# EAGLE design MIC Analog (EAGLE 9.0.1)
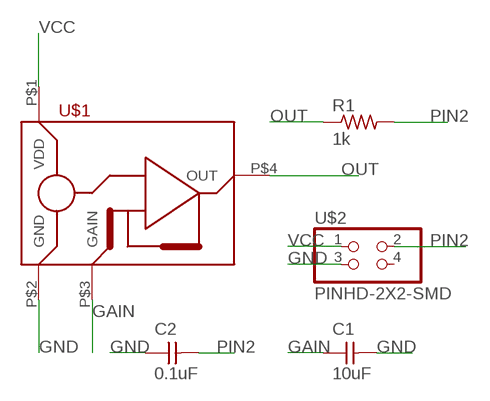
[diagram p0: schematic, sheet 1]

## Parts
C1  10uF  CAP-UNPOLARIZEDFAB  [C1206FAB]
C2  0.1uF  CAP-UNPOLARIZEDFAB  [C1206FAB]
R1  1k  RES-US1206FAB  [R1206FAB]
U$1  MEMS_MIC_SPU0414HR5H-SB  [CSP-4PIN]
U$2  PINHD-2X2-SMD  [2X02SMD]

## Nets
GAIN: C1.1 U$1.P$3(GAIN)
GND: C1.2 C2.1 U$1.P$2(GND) U$2.3
OUT: R1.1 U$1.P$4(OUT)
PIN2: C2.2 R1.2 U$2.2
VCC: U$1.P$1(VDD) U$2.1
Unconnected: U$2.4

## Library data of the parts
C1 C2 = fab:CAP-UNPOLARIZED
R1 = fab:RES-US: Resistor (US Symbol)
U$1 = fab:MEMS_MIC_SPU0414HR5H-SB
U$2 = fab:PINHD-2X2-SMD

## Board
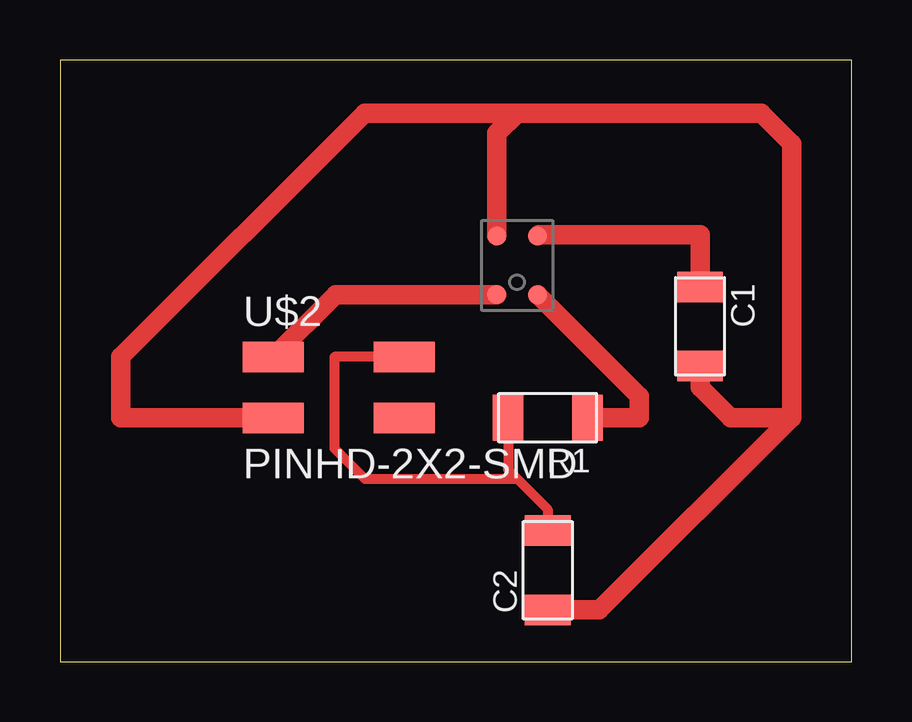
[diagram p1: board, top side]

Size 33 x 25.07 mm. Coordinates in mm from the lower left corner, seen from the top.
Outline: 0,0 33,0 33,25.07 0,25.07 0,0
Copper layers (1*16): Top 0.035mm / dielectric 1.5mm / Bottom 0.035mm
Design rules "default": minimum track width 6mil, minimum drill 0.35mm, track to track 6mil, track to pad 6mil, pad to pad 6mil, via to via 6mil, smd to smd 6mil, copper to edge 40mil, drill to drill 6mil, minimum pad ring 10mil, minimum via ring 8mil, stop-mask expansion 4mil, vias tented up to drill 0mil, thermal gap 10mil

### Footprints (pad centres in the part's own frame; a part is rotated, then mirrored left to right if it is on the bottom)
C1206FAB = smd 1.27 x 1.905: 1 -1.651,0; 2 1.651,0
R1206FAB = smd 1.27 x 1.905: 1 -1.651,0; 2 1.651,0
CSP-4PIN = smd 0.8 x 0.8: P$1 0.855,1.215; P$2 0.85,-1.23; P$3 -0.85,-1.23; P$4 -0.85,1.23
2X02SMD = smd 2.54 x 1.27: 1 -2.54,1.27; 2 2.92,1.27; 3 -2.54,-1.27; 4 2.92,-1.27

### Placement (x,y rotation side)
C1  26.67,13.97 270 top
C2  20.32,3.81 90 top
R1  20.32,10.16 180 top
U$1  19.05,16.51 180 top
U$2  11.43,11.43 0 top

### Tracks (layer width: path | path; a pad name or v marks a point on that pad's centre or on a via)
GAIN
  Top 0.813: U$1.P$3 19.94,17.78 26.67,17.78 C1.1
GND
  Top 0.813: U$1.P$2 18.2,22.01 19.05,22.86 | 19.05,22.86 29.21,22.86 30.48,21.59 30.48,10.16 | 30.48,10.16 27.94,10.16 26.67,11.43 C1.2 | 19.05,22.86 12.7,22.86 2.54,12.7 2.54,10.16 U$2.3 | C2.1 22.48,2.16 30.48,10.16
OUT
  Top 0.813: U$1.P$4 24.13,11.05 24.13,10.16 R1.1
PIN2
  Top 0.406: R1.2 18.67,8 19.05,7.62 | 19.05,7.62 20.32,6.35 C2.2 | U$2.2 11.43,12.7 11.43,8.89 12.7,7.62 19.05,7.62
VCC
  Top 0.813: U$1.P$1 11.48,15.3 U$2.1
